(* Logix 5000 AddOnInstructionDefinition export NXEE2_Program_Setup; software revision 20.05 *)

TYPE AMCI_NXEE2_Input_Data :
STRUCT
   Word_0_Reserved_Bit_0 : BOOL;
   Word_0_Reserved_Bit_1 : BOOL;
   CH1_Motion_Detection : BOOL;
   CH1_Velocity_at_Zero : BOOL;
   CH1_Command_Error : BOOL;
   CH1_Config_Error : BOOL;
   CH1_SSI_Setup_Error : BOOL;
   CH1_Scalar_Errors : BOOL;
   CH1_Preset_Value_Error : BOOL;
   CH1_FSC_Error : BOOL;
   CH1_FSC_Exceeded : BOOL;
   Memory_Error : BOOL;
   CH1_Input_State : BOOL;
   CH1_Value_Captured : BOOL;
   Heartbeat : BOOL;
   Acknowledge_Bit : BOOL;
   Word_1_Reserved_Bit_0 : BOOL;
   Word_1_Reserved_Bit_1 : BOOL;
   CH2_Motion_Detection : BOOL;
   CH2_Velocity_at_Zero : BOOL;
   CH2_Command_Error : BOOL;
   CH2_Config_Error : BOOL;
   CH2_SSI_Setup_Error : BOOL;
   CH2_Scalar_Errors : BOOL;
   CH2_Preset_Value_Error : BOOL;
   CH2_FSC_Error : BOOL;
   CH2_FSC_Exceeded : BOOL;
   Word_1_Reserved_bit_11 : BOOL;
   CH2_Input_State : BOOL;
   CH2_Value_Captured : BOOL;
   Word_1_Reserved_bit_14 : BOOL;
   Word_1_Reserved_bit_15 : BOOL;
   CH1_Value_1 : DINT;
   CH1_Value_2 : DINT;
   CH2_Value_1 : DINT;
   CH2_Value_2 : DINT;
END_STRUCT
END_TYPE

TYPE AMCI_NXEE2_Output_Data :
STRUCT
   Command_Word : INT;
   Configuration_Word : INT;
   Number_of_SSI_Data_Bits : INT;
   Number_Of_Data_Value_Bits : SINT;
   MSB_Number : SINT;
   Scalar_Multiplier : INT;
   Scalar_Divisor : INT;
   Preset_Value : DINT;
   Full_Scale_Count : DINT;
END_STRUCT
END_TYPE

ADD_ON_INSTRUCTION NXEE2_Program_Setup   (* revision 2.0, ExecuteEnableInFalse *)
// Revision note:
// 4/6/2021  Revision 1.0:.  Initial release
// 12/18/2025: Revision 2.0.  Modified the AOIs to use User Defined Input and Output Data.  Also, one setup AOI is now used for both channels.
VAR_IN_OUT
   NXEE2_Input_Data : AMCI_NXEE2_Input_Data; {required}
        .4   // command error
        .5   // config error
        .6   // setup error
        .7   // scalars errors
        .8   // preset value error
        .9   // full scale count error
   NXEE2_Output_Data : AMCI_NXEE2_Output_Data; {required}
END_VAR
VAR_INPUT
   Program_Channel_Number_1_or_2 : INT; {required}
   Network_input_data_format : INT; {required}
   Input_function : INT; {required}
   data_logic_0_positive_1_negative : BOOL; {required}
   data_type_0_binary_1_gray_code : BOOL; {required}
   count_direction_0_normal_1_reverse : BOOL; {required}
   velocity_update_0_160ms_1_24ms : BOOL; {required}
   SSI_Clock_Frequency : INT; {required}
   LED_0_enable_1_disable : BOOL; {required}
   Swap_32_bit_words_endian_0_NO_1_YES : BOOL; {required}
   save_in_flash_0_NO_1_YES : BOOL; {required}
   Number_of_SSI_Clock_Bits : INT; {required}
   MSB_Number : INT; {required}
   Number_of_Data_Value_Bits : INT; {required}
   Scalar_Multiplier : INT; {required}
   Scalar_Divisor : INT; {required}
   Preset_Value : DINT; {required}
   Full_Scale_Count : DINT; {required}
END_VAR
VAR_OUTPUT
   EN : BOOL; {access Read Only, visible}
   DN : BOOL; {access Read Only, visible}
   ER : BOOL; {access Read Only, visible}
END_VAR
VAR
   allow_programming : BOOL;
   command_data_block : INT[10];
        [0].0   // program channel 1
        [0].1   // program channel 2
        [0].2   // program ch0
        [0].4   // change channel 1 display format
        [0].5   // change channel 2 display format
        [0].14   // save in flash
        [0].15   // transmit bit
   internal_preset_value : DINT; {access None}
END_VAR

ROUTINE EnableInFalse   (* ladder *)
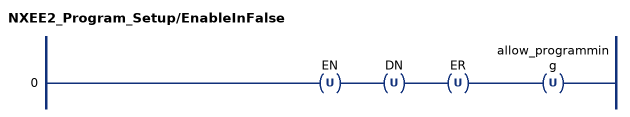
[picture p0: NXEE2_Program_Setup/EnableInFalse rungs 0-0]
   0: OTU(EN)OTU(DN)OTU(ER)OTU(allow_programming);
END_ROUTINE

ROUTINE Logic   (* ladder *)
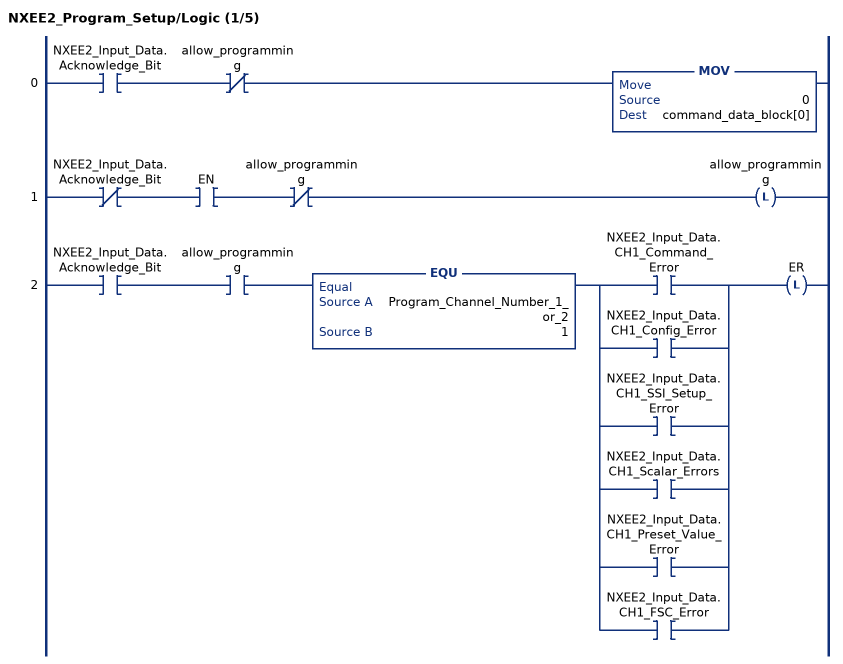
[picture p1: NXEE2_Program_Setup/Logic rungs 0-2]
   0: XIC(NXEE2_Input_Data.Acknowledge_Bit)XIO(allow_programming)MOV(0,command_data_block[0]);
   1: XIO(NXEE2_Input_Data.Acknowledge_Bit)XIC(EN)XIO(allow_programming)OTL(allow_programming);
   2: XIC(NXEE2_Input_Data.Acknowledge_Bit)XIC(allow_programming)EQU(Program_Channel_Number_1_or_2,1)[XIC(NXEE2_Input_Data.CH1_Command_Error) ,XIC(NXEE2_Input_Data.CH1_Config_Error) ,XIC(NXEE2_Input_Data.CH1_SSI_Setup_Error) ,XIC(NXEE2_Input_Data.CH1_Scalar_Errors) ,XIC(NXEE2_Input_Data.CH1_Preset_Value_Error) ,XIC(NXEE2_Input_Data.CH1_FSC_Error) ]OTL(ER);
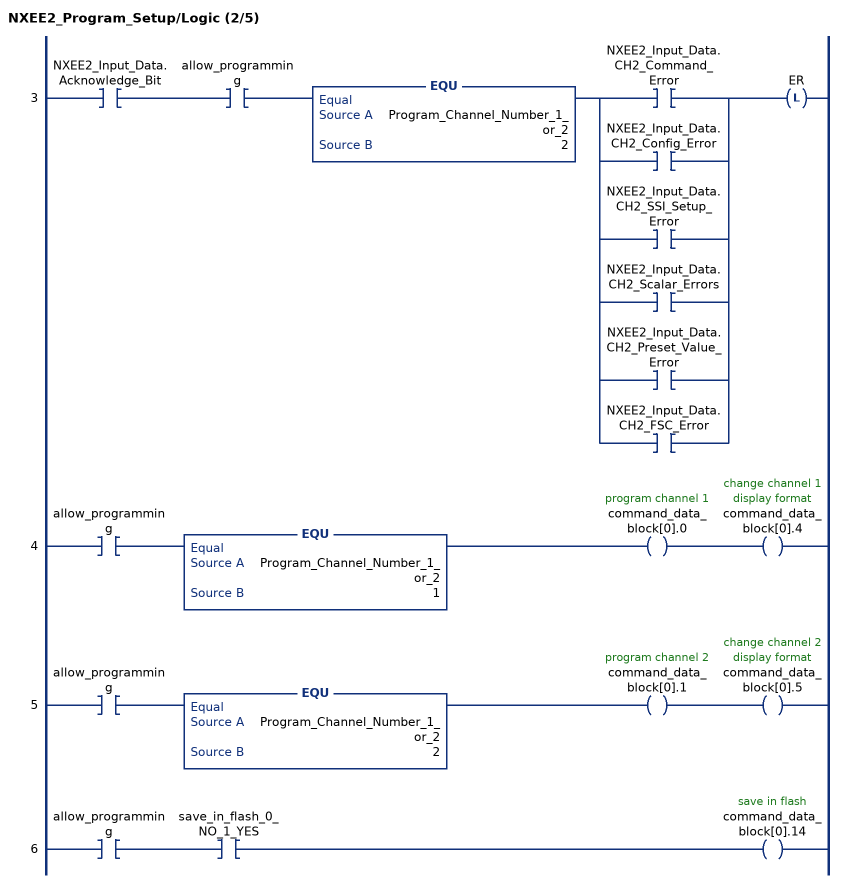
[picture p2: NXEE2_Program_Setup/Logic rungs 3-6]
   3: XIC(NXEE2_Input_Data.Acknowledge_Bit)XIC(allow_programming)EQU(Program_Channel_Number_1_or_2,2)[XIC(NXEE2_Input_Data.CH2_Command_Error) ,XIC(NXEE2_Input_Data.CH2_Config_Error) ,XIC(NXEE2_Input_Data.CH2_SSI_Setup_Error) ,XIC(NXEE2_Input_Data.CH2_Scalar_Errors) ,XIC(NXEE2_Input_Data.CH2_Preset_Value_Error) ,XIC(NXEE2_Input_Data.CH2_FSC_Error) ]OTL(ER);
   4: XIC(allow_programming)EQU(Program_Channel_Number_1_or_2,1)OTE(command_data_block[0].0)OTE(command_data_block[0].4);
   5: XIC(allow_programming)EQU(Program_Channel_Number_1_or_2,2)OTE(command_data_block[0].1)OTE(command_data_block[0].5);
   6: XIC(allow_programming)XIC(save_in_flash_0_NO_1_YES)OTE(command_data_block[0].14);
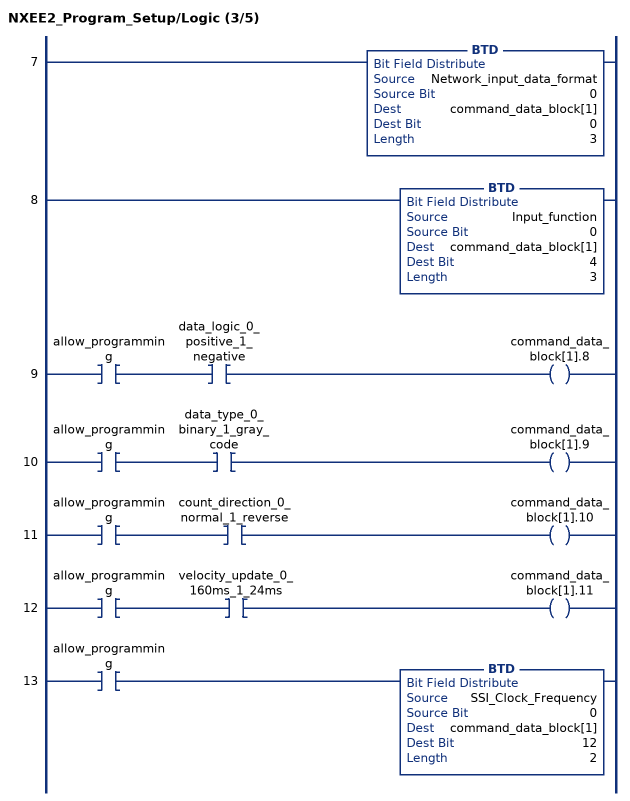
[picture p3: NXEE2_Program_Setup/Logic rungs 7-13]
   7: BTD(Network_input_data_format,0,command_data_block[1],0,3);
   8: BTD(Input_function,0,command_data_block[1],4,3);
   9: XIC(allow_programming)XIC(data_logic_0_positive_1_negative)OTE(command_data_block[1].8);
   10: XIC(allow_programming)XIC(data_type_0_binary_1_gray_code)OTE(command_data_block[1].9);
   11: XIC(allow_programming)XIC(count_direction_0_normal_1_reverse)OTE(command_data_block[1].10);
   12: XIC(allow_programming)XIC(velocity_update_0_160ms_1_24ms)OTE(command_data_block[1].11);
   13: XIC(allow_programming)BTD(SSI_Clock_Frequency,0,command_data_block[1],12,2);
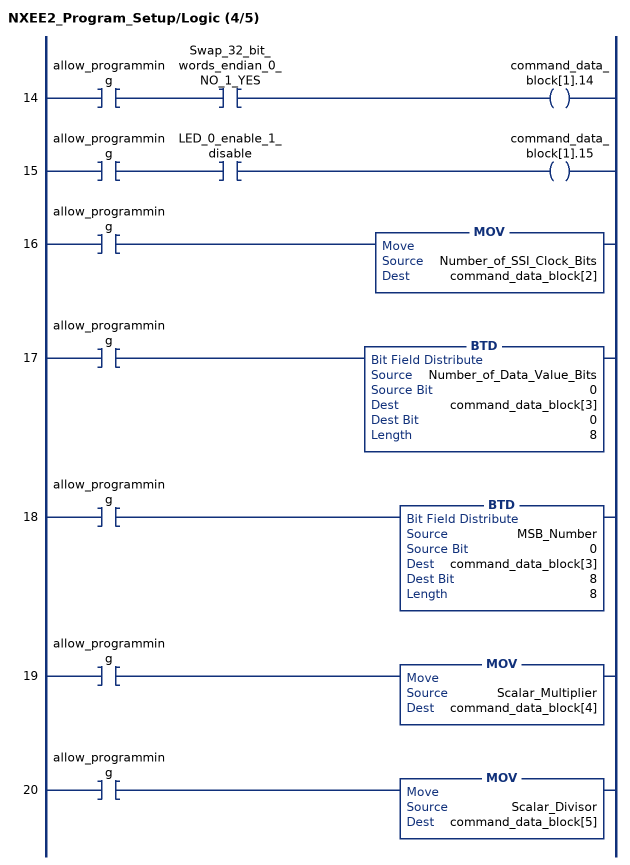
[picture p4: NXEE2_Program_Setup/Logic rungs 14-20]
   14: XIC(allow_programming)XIC(Swap_32_bit_words_endian_0_NO_1_YES)OTE(command_data_block[1].14);
   15: XIC(allow_programming)XIC(LED_0_enable_1_disable)OTE(command_data_block[1].15);
   16: XIC(allow_programming)MOV(Number_of_SSI_Clock_Bits,command_data_block[2]);
   17: XIC(allow_programming)BTD(Number_of_Data_Value_Bits,0,command_data_block[3],0,8);
   18: XIC(allow_programming)BTD(MSB_Number,0,command_data_block[3],8,8);
   19: XIC(allow_programming)MOV(Scalar_Multiplier,command_data_block[4]);
   20: XIC(allow_programming)MOV(Scalar_Divisor,command_data_block[5]);
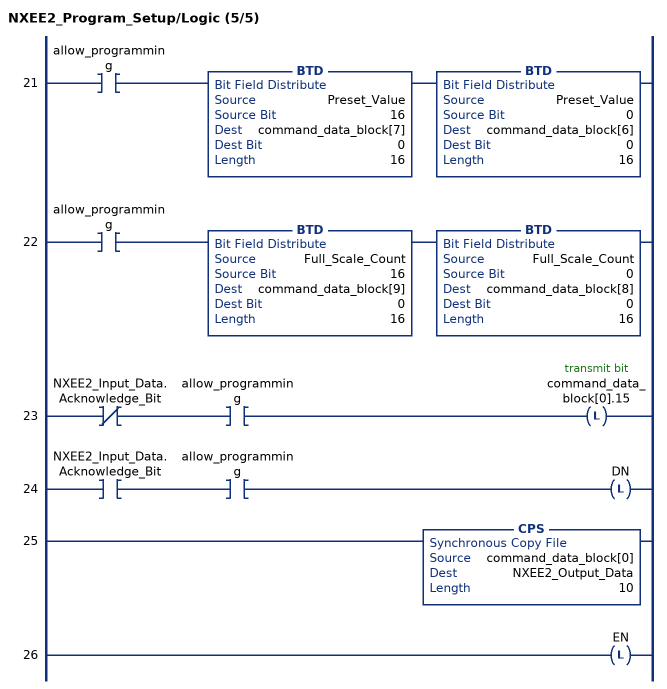
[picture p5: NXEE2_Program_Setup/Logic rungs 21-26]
   21: XIC(allow_programming)BTD(Preset_Value,16,command_data_block[7],0,16)BTD(Preset_Value,0,command_data_block[6],0,16);
   22: XIC(allow_programming)BTD(Full_Scale_Count,16,command_data_block[9],0,16)BTD(Full_Scale_Count,0,command_data_block[8],0,16);
   23: XIO(NXEE2_Input_Data.Acknowledge_Bit)XIC(allow_programming)OTL(command_data_block[0].15);
   24: XIC(NXEE2_Input_Data.Acknowledge_Bit)XIC(allow_programming)OTL(DN);
   25: CPS(command_data_block[0],NXEE2_Output_Data,10);
   26: OTL(EN);
END_ROUTINE
END_ADD_ON_INSTRUCTION
